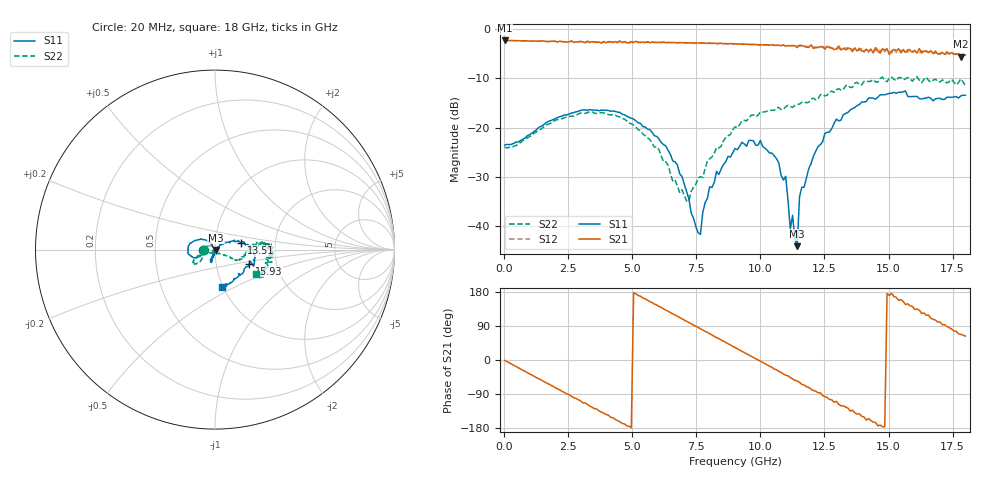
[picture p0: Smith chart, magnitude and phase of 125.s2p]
!Agilent Technologies,N5230A,US43500223,A.07.50.48
!Agilent N5230A: A.07.50.48
!Date: Sunday, January 10, 2016 16:15:56
!Correction: S11(Full 2 Port(1,2))
!S21(Full 2 Port(1,2))
!S12(Full 2 Port(1,2))
!S22(Full 2 Port(1,2))
!S2P File: Measurements: S11, S21, S12, S22:
# Hz S  RI  R 50
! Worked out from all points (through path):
!   201 points, 20 MHz to 18 GHz, reference 50 ohm
!   highest |S21| = -2.27 dB at 20 MHz (marker M1); lowest = -5.5 dB at 17.82 GHz (marker M2)
!   group delay of S21, straight-line fit = 101 ps
!   lowest |S11| = -44.1 dB at 11.44 GHz (marker M3), VSWR 1.01, Z = 50.6 - j0.256 ohm
!   |S11| at or under -10 dB: start of sweep to end of sweep
!   |S22| runs from -34.9 to -9.6 dB; largest |S21 - S12| = 0.078
!   S11 on the Smith chart (normalised r, x): 20 MHz: 0.88, +0.00; 13.51 GHz: 1.34, +0.10; 15.93 GHz: 1.45, -0.24; 18 GHz: 0.98, -0.43
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2e7  -0.0665 0.000284  0.7695 -0.011  0.7698 -0.0122  -0.0636 5.51e-07
1.5483e9  -0.0981 -0.0435  0.4169 -0.6385  0.4145 -0.6371  -0.0799 -0.063
3.0766e9  -0.1494 -0.0225  -0.2938 -0.6827  -0.2818 -0.6861  -0.1141 -0.0808
4.515e9  -0.1384 0.0359  -0.7223 -0.2216  -0.7353 -0.2074  -0.1159 -0.0541
6.0433e9  -0.0545 0.0541  -0.5768 0.4617  -0.5646 0.4603  -0.0555 -0.0218
7.1221e9  -0.0124 0.0186  -0.1536 0.7135  -0.1505 0.7145  -0.000636 -0.0179
7.6615e9  -0.00787 -0.00225  0.0967 0.7182  0.0977 0.7189  0.0229 -0.0218
8.0211e9  -0.0104 -0.0227  0.255 0.6803  0.2573 0.6729  0.0391 -0.0281
9.01e9  -0.0158 -0.0592  0.5941 0.3898  0.5962 0.3834  0.0889 -0.0495
1.06282e10  -0.0197 -0.0442  0.6188 -0.3004  0.6137 -0.3069  0.15 -0.0517
1.09878e10  -0.00794 -0.031  0.5139 -0.4342  0.5214 -0.4366  0.1576 -0.0415
1.11676e10  -0.0012 -0.00924  0.4691 -0.4917  0.4681 -0.4962  0.1614 -0.0298
1.12575e10  0.00866 -0.00943  0.4425 -0.5199  0.4388 -0.5217  0.1593 -0.0193
1.14373e10  0.00568 -0.00253  0.3731 -0.5348  0.3729 -0.5642  0.1685 -0.0318
1.15272e10  0.0143 0.0137  0.3577 -0.5885  0.3391 -0.5846  0.1725 -0.0166
1.20666e10  0.0418 0.0293  0.1047 -0.6308  0.1166 -0.6542  0.1992 0.00213
1.3505e10  0.1465 0.0375  -0.4456 -0.4504  -0.4347 -0.475  0.2546 0.025
1.50333e10  0.2218 -0.0252  -0.5456 0.0936  -0.5814 0.0936  0.3214 0.00721
1.59323e10  0.1916 -0.0783  -0.4577 0.3626  -0.4358 0.4052  0.2944 -0.0393
1.66515e10  0.1379 -0.1427  -0.2085 0.5687  -0.2327 0.5454  0.2854 -0.0529
1.78202e10  0.0658 -0.1993  0.2008 0.4889  0.2083 0.4902  0.2728 -0.1527
1.8e10  0.0374 -0.2096  0.2482 0.4876  0.2648 0.4757  0.2292 -0.1361
